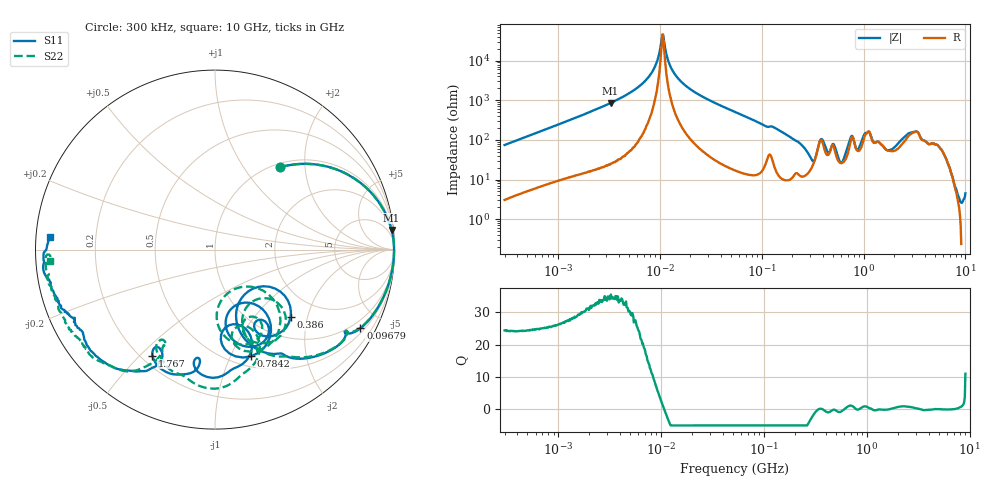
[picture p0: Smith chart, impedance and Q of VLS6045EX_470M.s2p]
! S-Parameter Data Generated by TDK Corporation
! Copyright(C) 2019 TDK Corporation.
! All Rights Reserved.
! TDK P/N: VLS6045EX-470M (Inductor)
! Property: L=47uH at 100kHz
! Size(LxWxT): 6x6x4.5mm
! Model Type: s2p (Touchstone File Format Version 1.0)
! Frequency: DC=Yes Start=0.3MHz Stop=10000MHz 802points Log-sweep
! Model Generated on May 10, 2019
! Port Assignments:
!  1 ---@@@--- 2
! Applicable Conditions:
!  Temperature = 25 degC
!  DC Bias Current = 0 A
!  Small Signal Operation
! Terms and conditions regarding TDK Simulation Models
! (1)This simulation model is being provided solely for informational purposes. Please refer to the specifications of the products in terms of detailed characteristics of such products.
! (2)In no event shall TDK Corporation of any of its subsidiaries be liable for any loss or damage arising, directly or indirectly,
!  From any information contained in this simulation model, including, but not limited to loss or damages arising from any inaccuracies, omissions or errors in connection with such information.
! (3)Any and all copyrights on this simulation model are owned by TDK Corporation.
!  Duplication or redistribution of this simulation model without prior written permission from TDK Corporation is prohibited.
! (4)This simulation model is subject to any modification or change without any prior notice.
! (5)Neither TDK Corporation nor any of its subsidiaries shall make any warranty, express or implied,
!  Including but not limited to the correctness, implied warranties of merchantability and fitness for a particular purpose with respect to this simulation models.
! (6)The use of this simulation model shall be deemed to have consented to the terms and conditions hereof.
# Hz S MA R 50
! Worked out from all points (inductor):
!   801 points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, 300 kHz to 10 GHz, reference 50 ohm
!   read as one part in series: L = 39.2 uH near 318.3 kHz
!   highest Q = 34.5 at 3.285 MHz (marker M1), where L = 41.2 uH
!   self-resonance near 10.62 MHz
!   S11 on the Smith chart (normalised r, x): 300 kHz: 1.07, +1.48; 96.79 MHz: 0.66, -3.84; 386 MHz: 1.43, -1.58; 784.2 MHz: 0.61, -1.20; 1.767 GHz: 0.24, -0.55; 10 GHz: 0.04, +0.04
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300000  0.5842 51.7  0.7878 -35.9  0.7882 -35.9  0.5839 51.7
1713600  0.9651 13.2  0.2317 -74.9  0.2317 -74.9  0.9651 13.2
3285409  0.9899 6.4  0.1163 -82.0  0.1163 -81.9  0.9899 6.4
6985119  0.9974 1.4  0.03492 -85.4  0.03492 -85.4  0.9975 1.4
9671944  0.9978 -0.4  0.008249 -75.8  0.008267 -75.7  0.9979 -0.4
1.07612e7  0.9978 -1.0  0.00218 11.7  0.002185 11.2  0.998 -0.9
1.273449e7  0.9975 -1.9  0.01399 78.6  0.01398 78.6  0.9977 -1.9
1.626666e7  0.9968 -3.4  0.03402 82.3  0.03403 82.3  0.997 -3.3
5.477226e7  0.9753 -15.8  0.1902 72.5  0.1902 72.5  0.9756 -15.5
9.679373e7  0.9211 -28.4  0.3412 58.7  0.3411 58.7  0.9221 -27.9
1.945824e8  0.7584 -53.2  0.5852 33.1  0.5852 33.1  0.7685 -51.4
3.126428e8  0.3827 -72.2  0.7643 -5.0  0.7644 -5.0  0.4136 -68.4
3.860116e8  0.5646 -41.8  0.4577 -14.4  0.4577 -14.4  0.5926 -49.9
5.344909e8  0.5703 -71.6  0.58 -14.2  0.5801 -14.2  0.547 -75.1
6.573376e8  0.3301 -67.5  0.7147 -45.5  0.7148 -45.5  0.2474 -69.4
7.84152e8  0.6277 -71.3  0.3745 -50.4  0.3745 -50.4  0.6135 -61.8
9.330971e8  0.4503 -70.8  0.5245 -71.1  0.5245 -71.1  0.4674 -66.9
1.180962e9  0.7021 -95.9  0.2712 -56.2  0.271 -56.2  0.7743 -92.4
1.767019e9  0.6861 -120.6  0.3483 -82.7  0.3477 -82.7  0.5827 -120.7
2.23379e9  0.7242 -116.7  0.2658 -127.1  0.2657 -127.1  0.6882 -117.7
3.34571e9  0.891 -143.4  0.06555 -121.8  0.06606 -121.4  0.9021 -137.5
1e10  0.9217 175.7  0.05513 -151.5  0.05489 -150.8  0.9206 -175.9
